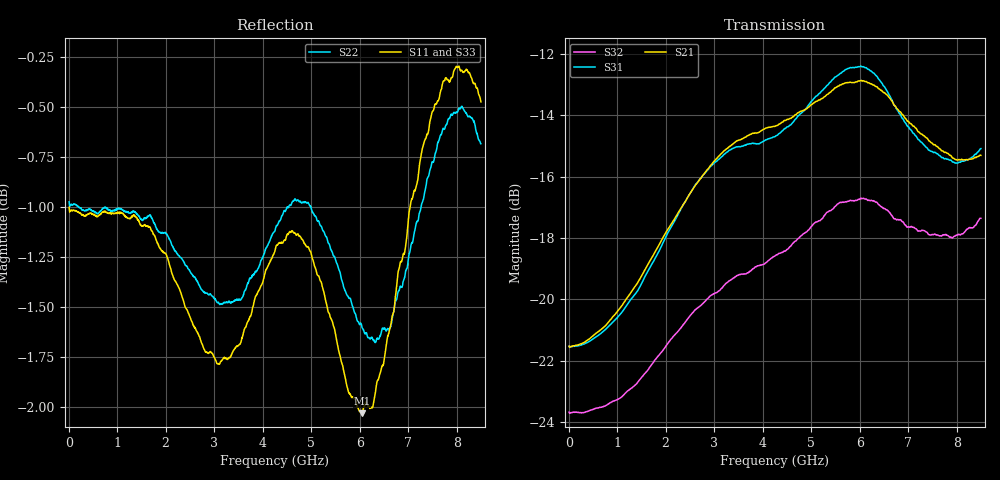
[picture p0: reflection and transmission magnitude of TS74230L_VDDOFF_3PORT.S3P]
!Agilent Technologies,E5071C,MY46522130,B.12.04
!Date: Fri Aug 01 10:38:32 2025
!Data & Calibration Information:
!Freq	S11:SOLT3(ON)	S13:SOLT3(ON)	S14:SOLT3(ON)
!	S31:SOLT3(ON)	S33:SOLT3(ON)	S34:SOLT3(ON)
!	S41:SOLT3(ON)	S43:SOLT3(ON)	S44:SOLT3(ON)
!PortZ  Port1:50+j0  Port3:50+j0  Port4:50+j0
!Above PortZ is port z conversion or system Z0 setting when saving the data.
!When reading, reference impedance value at option line is always used.
# Hz S dB R 50
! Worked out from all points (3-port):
!   1601 points, 10 MHz to 8.5 GHz, reference 50 ohm
!   strongest paths, dB at 10 MHz, 2.132 GHz, 4.255 GHz, 6.378 GHz, 8.5 GHz:
!     S21: -21.5, -17.5, -14.4, -13.1, -15.3
!     S31: -21.5, -17.6, -14.7, -12.8, -15.1
!     S32: -23.7, -21.3, -18.6, -16.9, -17.4
!   lowest |S11| = -2.0 dB at 6.049 GHz (marker M1), VSWR 8.60, Z = 71.9 + j154 ohm
!   |S11| at or under -10 dB: nowhere
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1e7  -1.00 179.4  -21.52 -0.4  -21.53 -0.4
     -21.53 -0.4  -0.97 179.4  -23.68 -0.5
     -21.52 -0.4  -23.68 -0.5  -0.97 179.4
1.055331e9  -1.03 159.2  -20.28 8.4  -20.50 7.5
            -20.29 8.4  -1.01 158.4  -23.22 -0.9
            -20.50 7.5  -23.22 -0.9  -0.99 158.6
2.036988e9  -1.25 142.2  -17.74 5.6  -17.85 5.6
            -17.74 5.5  -1.14 138.9  -21.44 -5.6
            -17.85 5.6  -21.46 -5.7  -1.17 140.7
3.209669e9  -1.75 105.4  -15.15 -13.4  -15.27 -15.4
            -15.15 -13.5  -1.48 111.1  -19.47 -23.3
            -15.27 -15.4  -19.54 -23.5  -1.50 107.6
4.255e9  -1.22 77.2  -14.36 -34.0  -14.69 -34.1
         -14.36 -34.1  -1.12 83.0  -18.64 -41.3
         -14.70 -34.2  -18.59 -41.1  -1.05 83.5
5.23135e9  -1.40 60.3  -13.44 -52.1  -13.20 -51.4
           -13.45 -52.2  -1.11 64.7  -17.33 -59.1
           -13.19 -51.4  -17.37 -59.2  -1.26 65.9
6.048512e9  -2.03 30.3  -12.86 -73.5  -12.41 -76.3
            -12.88 -73.6  -1.60 44.2  -16.66 -80.3
            -12.42 -76.3  -16.72 -80.5  -1.90 36.9
7.008944e9  -1.05 -2.4  -14.20 -98.1  -14.35 -102.1
            -14.21 -98.3  -1.25 12.4  -17.69 -102.5
            -14.38 -102.3  -17.64 -102.4  -1.14 2.9
7.741206e9  -0.37 -6.3  -15.18 -107.7  -15.44 -109.0
            -15.20 -107.9  -0.61 -3.3  -17.86 -112.3
            -15.42 -109.0  -17.90 -112.4  -0.56 -5.8
8.5e9  -0.48 -7.2  -15.31 -119.5  -15.04 -119.5
       -15.30 -119.5  -0.68 -16.0  -17.49 -128.1
       -15.09 -119.5  -17.36 -128.0  -0.84 -17.1
